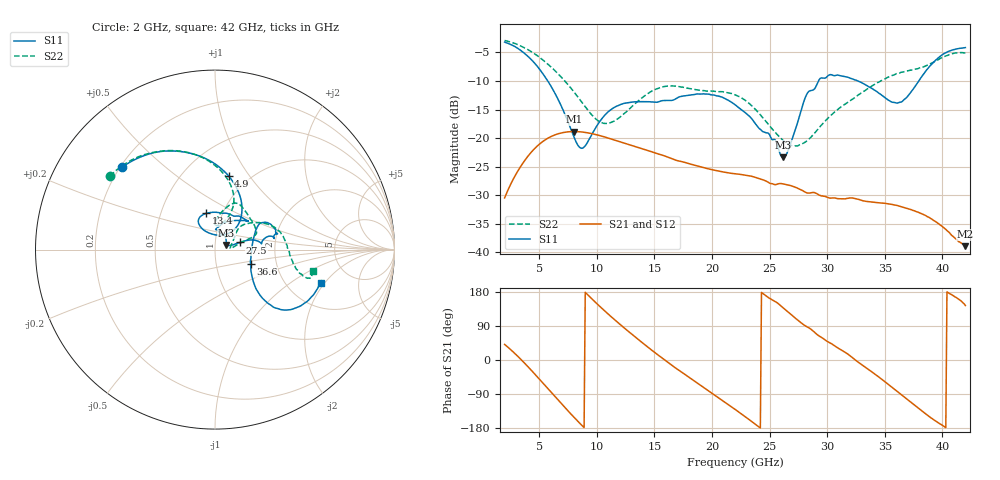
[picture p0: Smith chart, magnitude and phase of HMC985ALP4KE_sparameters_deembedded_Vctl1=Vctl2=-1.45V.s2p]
!s2p File: Measurements: S11, S21, S12, S22
# GHz S dB R 50.0
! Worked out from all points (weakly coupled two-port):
!   401 points, 2 GHz to 42 GHz, reference 50 ohm
!   highest |S21| = -18.85 dB at 8 GHz (marker M1); lowest = -38.9 dB at 42 GHz (marker M2)
!   lowest |S11| = -23.4 dB at 26.2 GHz (marker M3), VSWR 1.15, Z = 56.6 + j2.92 ohm
!   |S11| at or under -10 dB: 5.747 GHz to 29.25 GHz (23.5 GHz wide, 134 % of centre); 32.65 GHz to 37.95 GHz (5.298 GHz wide, 15 % of centre)
!   |S22| runs from -21.4 to -2.9 dB; largest |S21 - S12| = 0.00013
!   S11 on the Smith chart (normalised r, x): 2 GHz: 0.21, +0.36; 4.9 GHz: 0.81, +0.80; 13.4 GHz: 0.84, +0.36; 27.5 GHz: 1.32, +0.11; 36.6 GHz: 1.47, -0.24; 42 GHz: 3.07, -1.83
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2  -3.20 138.5  -30.45 41.1  -30.46 41.2  -2.91 145.1
3.4  -4.66 110.6  -24.94 2.0  -24.94 2.0  -3.88 121.9
4.9  -7.59 79.5  -21.26 -46.5  -21.27 -46.5  -5.67 98.3
6.2  -11.53 55.5  -19.57 -90.8  -19.58 -90.9  -7.87 80.6
8  -19.70 55.1  -18.85 -150.4  -18.86 -150.4  -11.87 67.1
8.7  -21.78 83.8  -18.93 -172.3  -18.93 -172.3  -13.72 67.5
10.8  -15.77 122.5  -19.87 126.4  -19.88 126.4  -17.44 86.3
13.4  -13.64 103.2  -21.51 59.2  -21.52 59.1  -13.84 81.6
15.4  -13.63 76.7  -22.81 11.4  -22.82 11.4  -11.22 68.8
18.9  -12.30 41.2  -24.97 -64.5  -24.97 -64.5  -11.61 42.5
22  -14.14 55.6  -26.23 -130.2  -26.24 -130.2  -12.42 19.9
24.5  -18.93 88.1  -27.35 173.7  -27.35 173.7  -16.61 14.5
26.2  -23.39 22.3  -28.02 137.1  -28.02 137.1  -20.45 5.6
27.5  -16.81 15.9  -28.84 103.9  -28.83 103.9  -21.28 7.6
28.2  -12.45 11.9  -29.55 88.4  -29.55 88.5  -20.55 15.9
28.7  -11.63 7.5  -29.52 78.6  -29.52 78.7  -19.59 22.4
31.1  -9.06 19.2  -30.61 28.7  -30.61 28.9  -14.70 42.2
33.3  -10.63 30.1  -31.02 -18.7  -31.04 -18.7  -11.67 34.9
35.4  -13.44 9.6  -31.53 -66.6  -31.52 -66.6  -9.27 22.4
36.6  -13.40 -21.8  -32.10 -95.3  -32.10 -95.3  -8.43 13.8
39.6  -6.04 -42.2  -34.88 -164.7  -34.88 -164.6  -6.32 -14.9
42  -4.16 -17.3  -38.91 143.8  -38.96 143.5  -5.09 -12.6
